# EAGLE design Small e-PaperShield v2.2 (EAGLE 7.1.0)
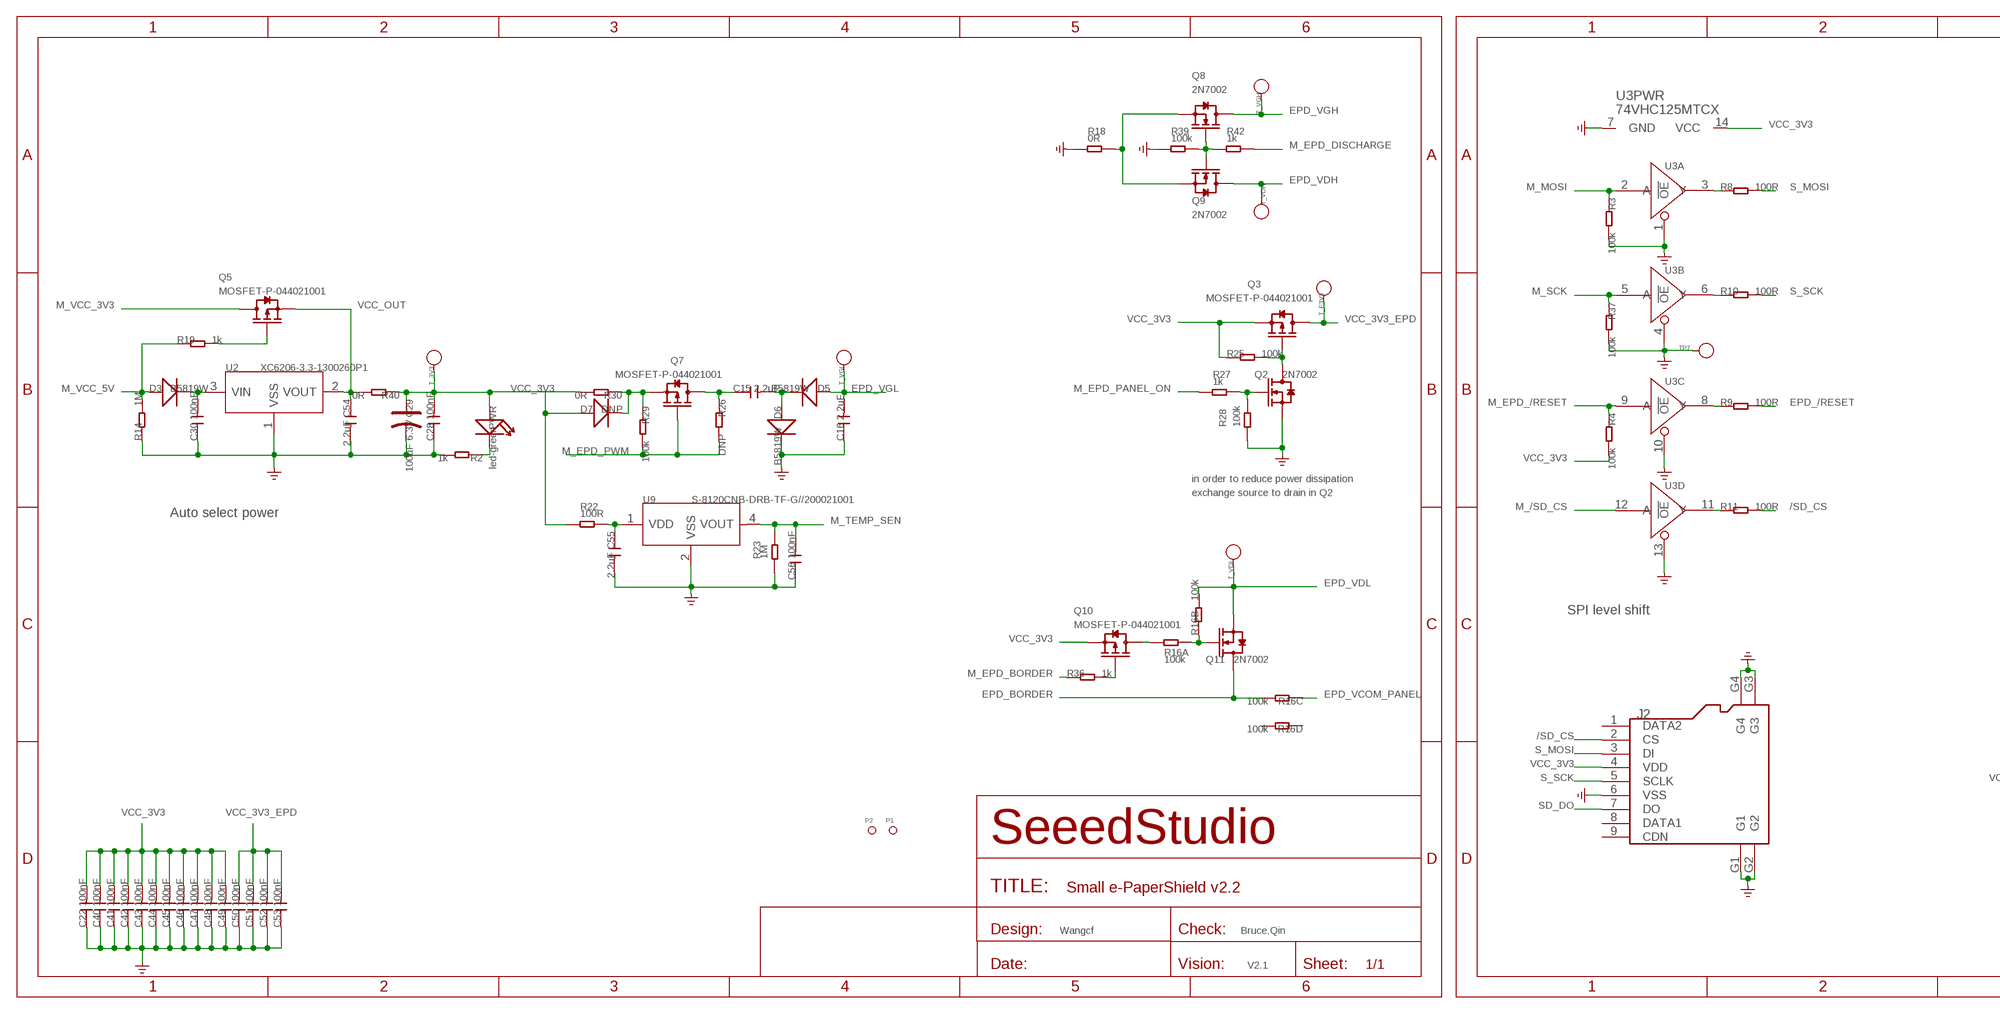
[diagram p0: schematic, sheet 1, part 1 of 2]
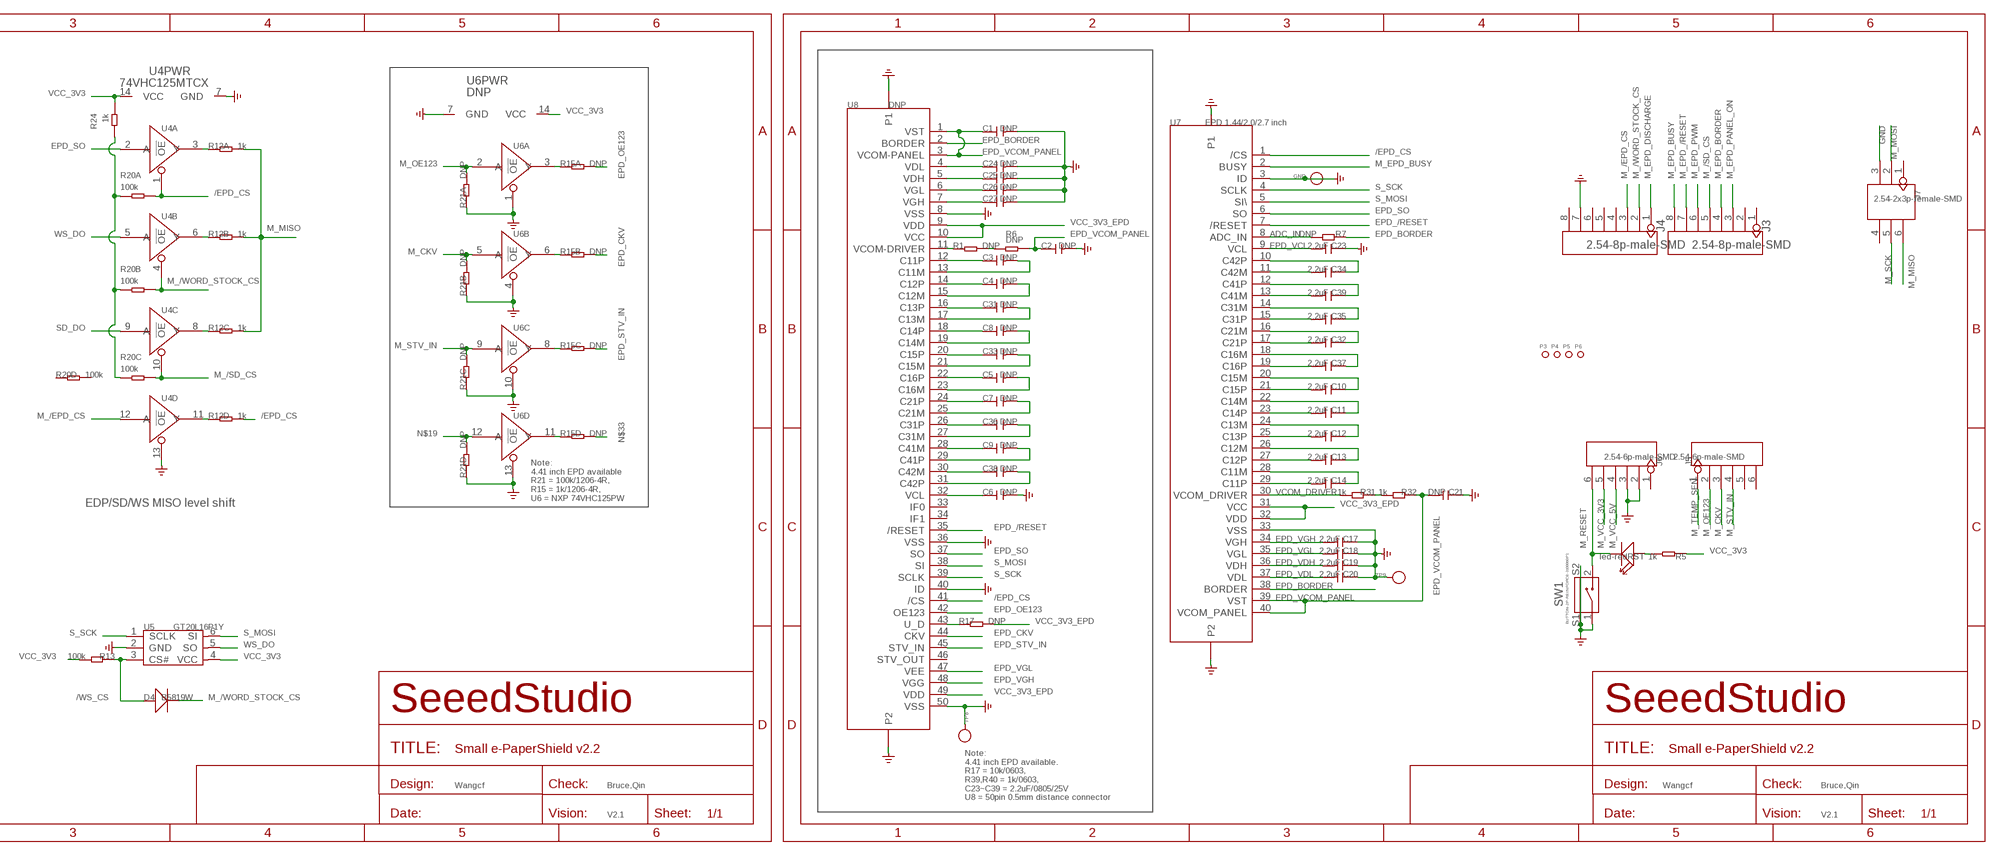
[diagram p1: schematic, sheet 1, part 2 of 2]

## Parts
C1  DNP  C-0805  [C0805]
C2  DNP  C-0805  [C0805]
C3  DNP  C-0805  [C0805]
C4  DNP  C-0805  [C0805]
C5  DNP  C-0805  [C0805]
C6  DNP  C-0805  [C0805]
C7  DNP  C-0805  [C0805]
C8  DNP  C-0805  [C0805]
C9  DNP  C-0805  [C0805]
C10  2.2uF  C-0805  [C0805]
C11  2.2uF  C-0805  [C0805]
C12  2.2uF  C-0805  [C0805]
C13  2.2uF  C-0805  [C0805]
C14  2.2uF  C-0805  [C0805]
C15  2.2uF  C-0805  [C0805]
C16  2.2uF  C-0805  [C0805]
C17  2.2uF  C-0805  [C0805]
C18  2.2uF  C-0805  [C0805]
C19  2.2uF  C-0805  [C0805]
C20  2.2uF  C-0805  [C0805]
C21  DNP  C-0805  [C0805]
C22  100nF  C-0603  [C0603]
C23  2.2uF  C-0805  [C0805]
C24  DNP  C-0805  [C0805]
C25  DNP  C-0805  [C0805]
C26  DNP  C-0805  [C0805]
C27  DNP  C-0805  [C0805]
C28  100nF  C-0603  [C0603]
C29  100uF 6.3V  CAP-AVX-B  [AVX-B]
C30  100nF  C-0603  [C0603]
C31  DNP  C-0805  [C0805]
C32  2.2uF  C-0805  [C0805]
C33  DNP  C-0805  [C0805]
C34  2.2uF  C-0805  [C0805]
C35  2.2uF  C-0805  [C0805]
C36  DNP  C-0805  [C0805]
C37  2.2uF  C-0805  [C0805]
C38  DNP  C-0805  [C0805]
C39  2.2uF  C-0805  [C0805]
C40  100nF  C-0603  [C0603]
C41  100nF  C-0603  [C0603]
C42  100nF  C-0603  [C0603]
C43  100nF  C-0603  [C0603]
C44  100nF  C-0603  [C0603]
C45  100nF  C-0603  [C0603]
C46  100nF  C-0603  [C0603]
C47  100nF  C-0603  [C0603]
C48  100nF  C-0603  [C0603]
C49  100nF  C-0603  [C0603]
C50  100nF  C-0603  [C0603]
C51  100nF  C-0603  [C0603]
C52  100nF  C-0603  [C0603]
C53  100nF  C-0603  [C0603]
C54  2.2uF  C-0805  [C0805]
C55  2.2uF  C-0805  [C0805]
C56  100nF  C-0603  [C0603]
D3  B5819W  D'1206'  [SOD123]
D4  B5819W  D'1206'  [SOD123]
D5  B5819W  D'1206'  [SOD123]
D6  B5819W  D'1206'  [SOD123]
D7  DNP  D'1206'  [SOD123]
GND  PAD-TEST-POINT'3535'  [TP_3535]
J2  HOLDER-MICROSD-9P  [9P-SMD-W/-RING]
J3  2.54-8p-male-SMD  HEADER-8P-2.54-SMD  [8P-2.54-SMD]
J4  2.54-8p-male-SMD  HEADER-8P-2.54-SMD  [8P-2.54-SMD]
J5  2.54-6p-male-SMD  HEADER-6P-SMD  [6P-2.54-SMD]
J6  2.54-6p-male-SMD  HEADER-6P-SMD  [6P-2.54-SMD]
J7  2.54-2x3p-female-SMD  HEADER-2X3P-SMD  [2X3P-2.54-SMD]
P1  PAD-MARK'ANNULAR'  [ROUND-MARK-1.0]
P2  PAD-MARK'ANNULAR'  [ROUND-MARK-1.0]
P3  PAD-MARK'ANNULAR'  [ROUND-MARK-1.0]
P4  PAD-MARK'ANNULAR'  [ROUND-MARK-1.0]
P5  PAD-MARK'ANNULAR'  [ROUND-MARK-1.0]
P6  PAD-MARK'ANNULAR'  [ROUND-MARK-1.0]
PWR  led-green  LED'RIGHT'  [LED-SIDE-VIEW-0603-RIGHT]
Q2  2N7002  MOSFET-N'SOT23'  [SOT23]
Q3  MOSFET-P-044021001  [SOT23]
Q5  MOSFET-P-044021001  [SOT23]
Q7  MOSFET-P-044021001  [SOT23]
Q8  2N7002  MOSFET-N'SOT23'  [SOT23]
Q9  2N7002  MOSFET-N'SOT23'  [SOT23]
Q10  MOSFET-P-044021001  [SOT23]
Q11  2N7002  MOSFET-N'SOT23'  [SOT23]
R1  DNP  R-0603  [R0603]
R2  1k  R-0603  [R0603]
R3  100k  R-0603  [R0603]
R4  100k  R-0603  [R0603]
R5  1k  R-0603  [R0603]
R6  DNP  R-0603  [R0603]
R7  DNP  R-0603  [R0603]
R8  100R  R-0603  [R0603]
R9  100R  R-0603  [R0603]
R10  100R  R-0603  [R0603]
R11  100R  R-0603  [R0603]
R12  1k  R-4R-1206  [1206-8-3.3X2.4]
R13  100k  R-0603  [R0603]
R14  1M  R-0603  [R0603]
R15  DNP  R-4R-1206  [1206-8-3.3X2.4]
R16  100k  R-4R-1206  [1206-8-3.3X2.4]
R17  DNP  R-0603  [R0603]
R18  0R  R-0603  [R0603]
R19  1k  R-0603  [R0603]
R20  100k  R-4R-1206  [1206-8-3.3X2.4]
R21  DNP  R-4R-1206  [1206-8-3.3X2.4]
R22  100R  R-0603  [R0603]
R23  1M  R-0603  [R0603]
R24  1k  R-0603  [R0603]
R25  100k  R-0603  [R0603]
R26  DNP  R-0603  [R0603]
R27  1k  R-0603  [R0603]
R28  100k  R-0603  [R0603]
R29  100k  R-0603  [R0603]
R30  0R  R-0603  [R0603]
R31  1k  R-0603  [R0603]
R32  1k  R-0603  [R0603]
R36  1k  R-0603  [R0603]
R37  100k  R-0603  [R0603]
R39  100k  R-0603  [R0603]
R40  0R  R-0603  [R0603]
R42  1k  R-0603  [R0603]
RST  led-red  LED'RIGHT'  [LED-SIDE-VIEW-0603-RIGHT]
SW1  BUTTON-2P-REINFORCE-3100060P1  [4P-SMD-7.0X3.5X3.5H-90D]
T_3V3  PAD-TEST-POINT'3535'  [TP_3535]
T_E3V3  PAD-TEST-POINT'3535'  [TP_3535]
T_VDH  PAD-TEST-POINT'3535'  [TP_3535]
T_VDL  PAD-TEST-POINT'3535'  [TP_3535]
T_VGH  PAD-TEST-POINT'3535'  [TP_3535]
T_VGL  PAD-TEST-POINT'3535'  [TP_3535]
TP7  PAD-TEST-POINT'3535'  [TP_3535]
TP8  PAD-TEST-POINT'3535'  [TP_3535]
TP9  PAD-TEST-POINT'3535'  [TP_3535]
U2  XC6206-3.3-1300260P1  [SOT23]
U3  74VHC125MTCX  74VHC125PW  [TSSOP14]
U4  74VHC125MTCX  74VHC125PW  [TSSOP14]
U5  GT20L16P1Y  [SOT23-6]
U6  DNP  74VHC125PW  [TSSOP14]
U7  EPD 1.44/2.0/2.7 inch  TFT-EPD-PANEL  [40P-0.5]
U8  DNP  TFT-EPD-PANEL  [50P-0.5]
U9  S-8120CNB-DRB-TF-G//200021001  S-8110C/8120C  [SC-82AB]

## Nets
3V3_LOG: R20.1 R20.2 R20.3 R24.2
/EPD_CS: R12.5 R20.8 U4.1(A:!OE) U7.1(/CS) U8.41(/CS)
/SD_CS: J2.2(CS) R11.2
/WS_CS: D4.+ R13.1 U5.3(CS#)
ADC_IN: R7.2 U7.8(ADC_IN)
EPD_/RESET: R9.2 U7.7(/RESET) U8.35(/RESET)
EPD_BORDER: Q11.3(D) R7.1 R16.6 U7.38(BORDER) U8.2(BORDER)
EPD_CKV: R15.7 U8.44(CKV)
EPD_OE123: R15.8 U8.42(OE123)
EPD_SO: U4.2(A:A) U7.6(SO) U8.37(SO)
EPD_STV_IN: R15.6 U8.45(STV_IN)
EPD_VCL: C23.2 U7.9(VCL)
EPD_VCOM_PANEL: C1.1 C2.1 C21.2 R6.2 R16.3 R32.1 U7.39(VST) U7.40(VCOM_PANEL) U8.1(VST) U8.3(VCOM-PANEL)
EPD_VDH: C19.2 C25.1 Q9.3(D) T_VDH.T U7.36(VDH) U8.5(VDH)
EPD_VDL: C20.2 C24.1 Q11.2(S) R16.7 T_VDL.T U7.37(VDL) U8.4(VDL)
EPD_VGH: C17.2 C27.1 Q8.3(D) T_VGH.T U7.34(VGH) U8.7(VGH) U8.48(VGG)
EPD_VGL: C16.2 C18.2 C26.1 D5.+ T_VGL.T U7.35(VGL) U8.6(VGL) U8.47(VEE)
GND: C1.2 C2.2 C6.2 C16.1 C17.1 C18.1 C19.1 C20.1 C21.1 C22.1 C23.1 C24.2 C25.2 C26.2 C27.2 C28.1 C29.- C30.1 C40.1 C41.1 C42.1 C43.1 C44.1 C45.1 C46.1 C47.1 C48.1 C49.1 C50.1 C51.1 C52.1 C53.1 C54.2 C55.2 C56.1 D6.- GND.T J2.6(VSS) J2.G1 J2.G2 J2.G3 J2.G4 J4.7 J6.2 J6.3 J7.3 Q2.2(S) R2.2 R3.2 R14.1 R18.1 R21.1 R21.2 R21.3 R21.4 R23.1 R28.1 R37.2 R39.1 SW1.1 SW1.S1 SW1.S2 TP7.T TP8.T TP9.T U2.1(VSS) U3.1(A:!OE) U3.4(B:!OE) U3.7(PWR:GND) U3.10(C:!OE) U3.13(D:!OE) U4.7(PWR:GND) U4.13(D:!OE) U5.2(GND) U6.1(A:!OE) U6.4(B:!OE) U6.7(PWR:GND) U6.10(C:!OE) U6.13(D:!OE) U7.3(ID) U7.33(VSS) U7.P1 U7.P2 U8.8(VSS) U8.36(VSS) U8.40(ID) U8.50(VSS) U8.P1 U8.P2 U9.2(VSS)
M_/EPD_CS: J4.3 U4.12(D:A)
M_/SD_CS: J3.5 R20.6 U3.12(D:A) U4.10(C:!OE)
M_/WORD_STOCK_CS: D4.- J4.2 R20.7 U4.4(B:!OE)
M_CKV: J5.3 R21.7 U6.5(B:A)
M_EPD_/RESET: J3.7 R4.1 U3.9(C:A)
M_EPD_BORDER: J3.4 R36.1
M_EPD_BUSY: J3.8 U7.2(BUSY)
M_EPD_DISCHARGE: J4.1 R42.2
M_EPD_PANEL_ON: J3.3 R27.1
M_EPD_PWM: J3.6 Q7.1(G) R26.2 R29.2
M_MISO: J7.6 R12.6 R12.7 R12.8
M_MOSI: J7.2 R3.1 U3.2(A:A)
M_OE123: J5.2 R21.8 U6.2(A:A)
M_RESET: J6.6 RST.2(-) SW1.2
M_SCK: J7.5 R37.1 U3.5(B:A)
M_STV_IN: J5.4 R21.6 U6.9(C:A)
M_TEMP_SEN: C56.2 J5.1 R23.2 U9.4(VOUT)
M_VCC_3V3: J6.5 Q5.3(D)
M_VCC_5V: D3.+ J6.4 R14.2 R19.1
N$1: PWR.2(-) R2.1
N$2: Q5.1(G) R19.2
N$3: C15.2 D5.- D6.+
N$4: D7.- Q7.2(S) R29.1 R30.1
N$6: Q2.1(G) R27.2 R28.2
N$7: R11.1 U3.11(D:Y)
N$8: C30.2 D3.- U2.3(VIN)
N$9: C15.1 Q7.3(D) R26.1
N$10: Q8.1(G) Q9.1(G) R39.2 R42.1
N$11: Q2.3(D) Q3.1(G) R25.2
N$12: R31.1 R32.2
N$13: Q10.3(D) R16.1
N$14: Q10.1(G) R36.2
N$15: C4.1 U8.14(C12P)
N$16: Q8.2(S) Q9.2(S) R18.2
N$19: R21.5 U6.12(D:A)
N$20: R12.1 U4.3(A:Y)
N$21: R12.2 U4.6(B:Y)
N$22: R12.3 U4.8(C:Y)
N$23: R15.1 U6.3(A:Y)
N$24: R15.3 U6.8(C:Y)
N$25: R15.4 U6.11(D:Y)
N$26: R15.2 U6.6(B:Y)
N$27: R12.4 U4.11(D:Y)
N$28: Q11.1(G) R16.2 R16.8
N$30: R1.2 R6.1
N$33: R15.5
N$34: C34.1 U7.10(C42P)
N$35: C34.2 U7.11(C42M)
N$36: C39.1 U7.12(C41P)
N$37: C39.2 U7.13(C41M)
N$39: C4.2 U8.15(C12M)
N$40: C3.1 U8.12(C11P)
N$41: C31.2 U8.17(C13M)
N$42: C31.1 U8.16(C13P)
N$43: C8.1 U8.18(C14P)
N$44: C8.2 U8.19(C14M)
N$45: C33.2 U8.21(C15M)
N$46: C33.1 U8.20(C15P)
N$47: C5.1 U8.22(C16P)
N$48: C5.2 U8.23(C16M)
N$49: C7.1 U8.24(C21P)
N$50: C7.2 U8.25(C21M)
N$51: C36.1 U8.26(C31P)
N$52: C36.2 U8.27(C31M)
N$53: C9.1 U8.28(C41M)
N$54: C9.2 U8.29(C41P)
N$55: C38.1 U8.30(C42M)
N$56: C38.2 U8.31(C42P)
N$57: C6.1 U8.32(VCL)
N$58: R1.1 U8.11(VCOM-DRIVER)
N$67: R17.1 U8.43(U_D)
N$74: R8.1 U3.3(A:Y)
N$76: R10.1 U3.6(B:Y)
N$80: R9.1 U3.8(C:Y)
N$81: C35.1 U7.14(C31M)
N$82: C3.2 U8.13(C11M)
N$85: C35.2 U7.15(C31P)
N$87: R5.2 RST.1(+)
N$88: C32.1 U7.16(C21M)
N$89: C32.2 U7.17(C21P)
N$90: C37.1 U7.18(C16M)
N$91: C37.2 U7.19(C16P)
N$92: C10.1 U7.20(C15M)
N$93: C10.2 U7.21(C15P)
N$94: C11.1 U7.22(C14M)
N$95: C11.2 U7.23(C14P)
N$96: C12.1 U7.24(C13M)
N$97: C12.2 U7.25(C13P)
N$98: C13.1 U7.26(C12M)
N$99: C13.2 U7.27(C12P)
N$100: C14.1 U7.28(C11M)
N$101: C14.2 U7.29(C11P)
S_MOSI: J2.3(DI) R8.2 U5.6(SI) U7.5(SI\) U8.38(SI)
S_SCK: J2.5(SCLK) R10.2 U5.1(SCLK) U7.4(SCLK) U8.39(SCLK)
SD_DO: J2.7(DO) U4.9(C:A)
VCC_3V3: C22.2 C28.2 C29.+ C40.2 C41.2 C42.2 C43.2 C44.2 C45.2 C46.2 C47.2 C48.2 C49.2 D7.+ J2.4(VDD) PWR.1(+) Q3.2(S) Q10.2(S) R4.2 R5.1 R13.2 R22.1 R24.1 R25.1 R30.2 R40.1 T_3V3.T U3.14(PWR:VCC) U4.14(PWR:VCC) U5.4(VCC) U6.14(PWR:VCC)
VCC_3V3_EPD: C50.2 C51.2 C52.2 C53.2 Q3.3(D) R17.2 T_E3V3.T U7.31(VCC) U7.32(VDD) U8.9(VDD) U8.10(VCC) U8.49(VDD)
VCC_OUT: C54.1 Q5.2(S) R40.2 U2.2(VOUT)
VCOM_DRIVER: R31.2 U7.30(VCOM_DRIVER)
VDD: C55.1 R22.2 U9.1(VDD)
WS_DO: U4.5(B:A) U5.5(SO)
Unconnected: J2.1(DATA2) J2.8(DATA1) J2.9(CDN) J3.1 J3.2 J4.4 J4.5 J4.6 J4.8 J5.5 J5.6 J6.1 J7.1 J7.4 R16.4 R16.5 R20.4 R20.5 U8.33(IF0) U8.34(IF1) U8.46(STV_OUT)

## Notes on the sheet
- in order to reduce power dissipation
- exchange source to drain in Q2
- Auto select power
- Note:
  4.41 inch EPD available
  R21 = 100k/1206-4R,
  R15 = 1k/1206-4R,
  U6 = NXP 74VHC125PW
- EDP/SD/WS MISO level shift
- SPI level shift
- Wangcf | Bruce,Qin | Wangcf | Bruce,Qin | Wangcf | Bruce,Qin
- Note:
  4.41 inch EPD available.
  R17 = 10k/0603, 
  R39,R40 = 1k/0603, 
  C23~C39 = 2.2uF/0805/25V
  U8 = 50pin 0.5mm distance connector
- V2.1 | V2.1 | V2.1

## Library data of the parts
C1-C28 C30-C56 = Discrete:C*: Ceramic Capacitors
C29 = Discrete:CAP*: Electrolytic Capacitors,Tantalum Capacitors and Super Capacitors
D3-D7 = Discrete:D*
GND T_3V3 T_E3V3 T_VDH T_VDL T_VGH T_VGL TP7-TP9 = Discrete:PAD-TEST-POINT; PARTNO: DNP
J2 = Connector :HOLDER-MICROSD-9P
J3 J4 = Connector:HEADER-8P
J5 J6 = Connector:HEADER-6P
J7 = Connector:HEADER-2X3P
P1-P6 = Discrete:PAD-MARK; PARTNO: DNP
PWR RST = Discrete:LED*
Q2 Q8 Q9 Q11 = Discrete:MOSFET-N: IRLL014: http://www.vishay.com/docs/91319/sihll014.pdf
Q3 Q5 Q7 Q10 = OPL:MOSFET-P: CJ2305：SMD MOSFET P-CH 8V-4.1A
R1-R11 R13 R14 R17-R19 R22-R32 R36 R37 R39 R40 R42 = Discrete:R*
R12 R15 R16 R20 R21 = Discrete:R-4R*: Resistor Array
SW1 = Discrete:BUTTON-2P-REINFORCE: TS-1188E http://www.best-dz.com/?thread-374-2.html SMD Button
U2 = OPL:XC6206-3.3: LOW ESR Cap.Compatible Positive Voltage Regulators
U3 U4 U6 = IC:74V*125: Quad Buffer/Line Driver;3-state
U5 = template:GT20L16P1Y
U7 = moudle:TFT-EPD-PANEL: 1.44inch/2.0inch/2.7inch TFT EPD Panel
U8 = template:TFT-EPD-PANEL: 4.4inch TFT EPD PANEL
U9 = template:S-8110C/8120C: COMS Temperature Sensor IC

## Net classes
0 default: width 0.152 mm, drill 0.305 mm, clearance 0.152 mm

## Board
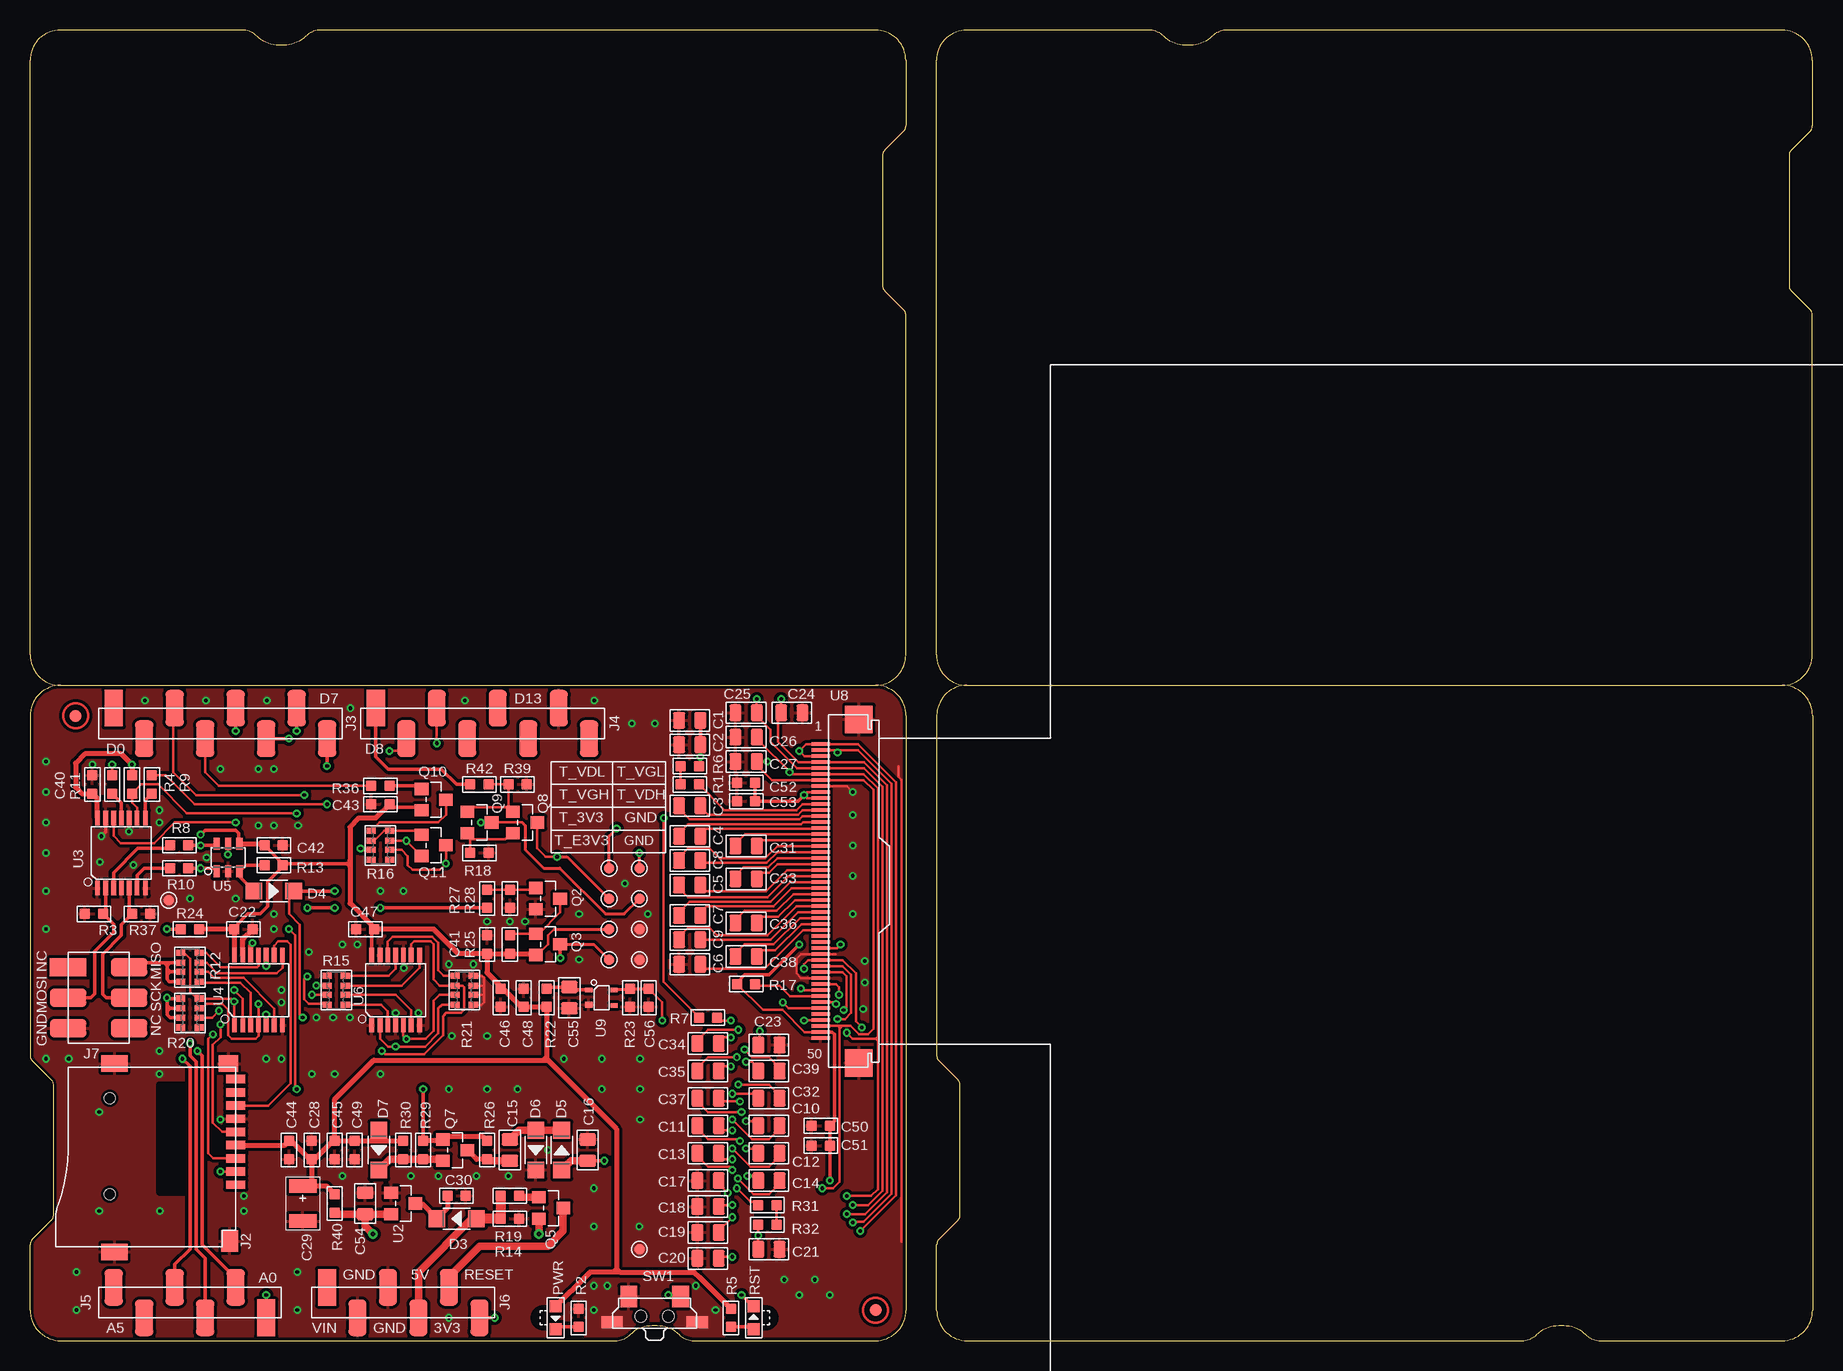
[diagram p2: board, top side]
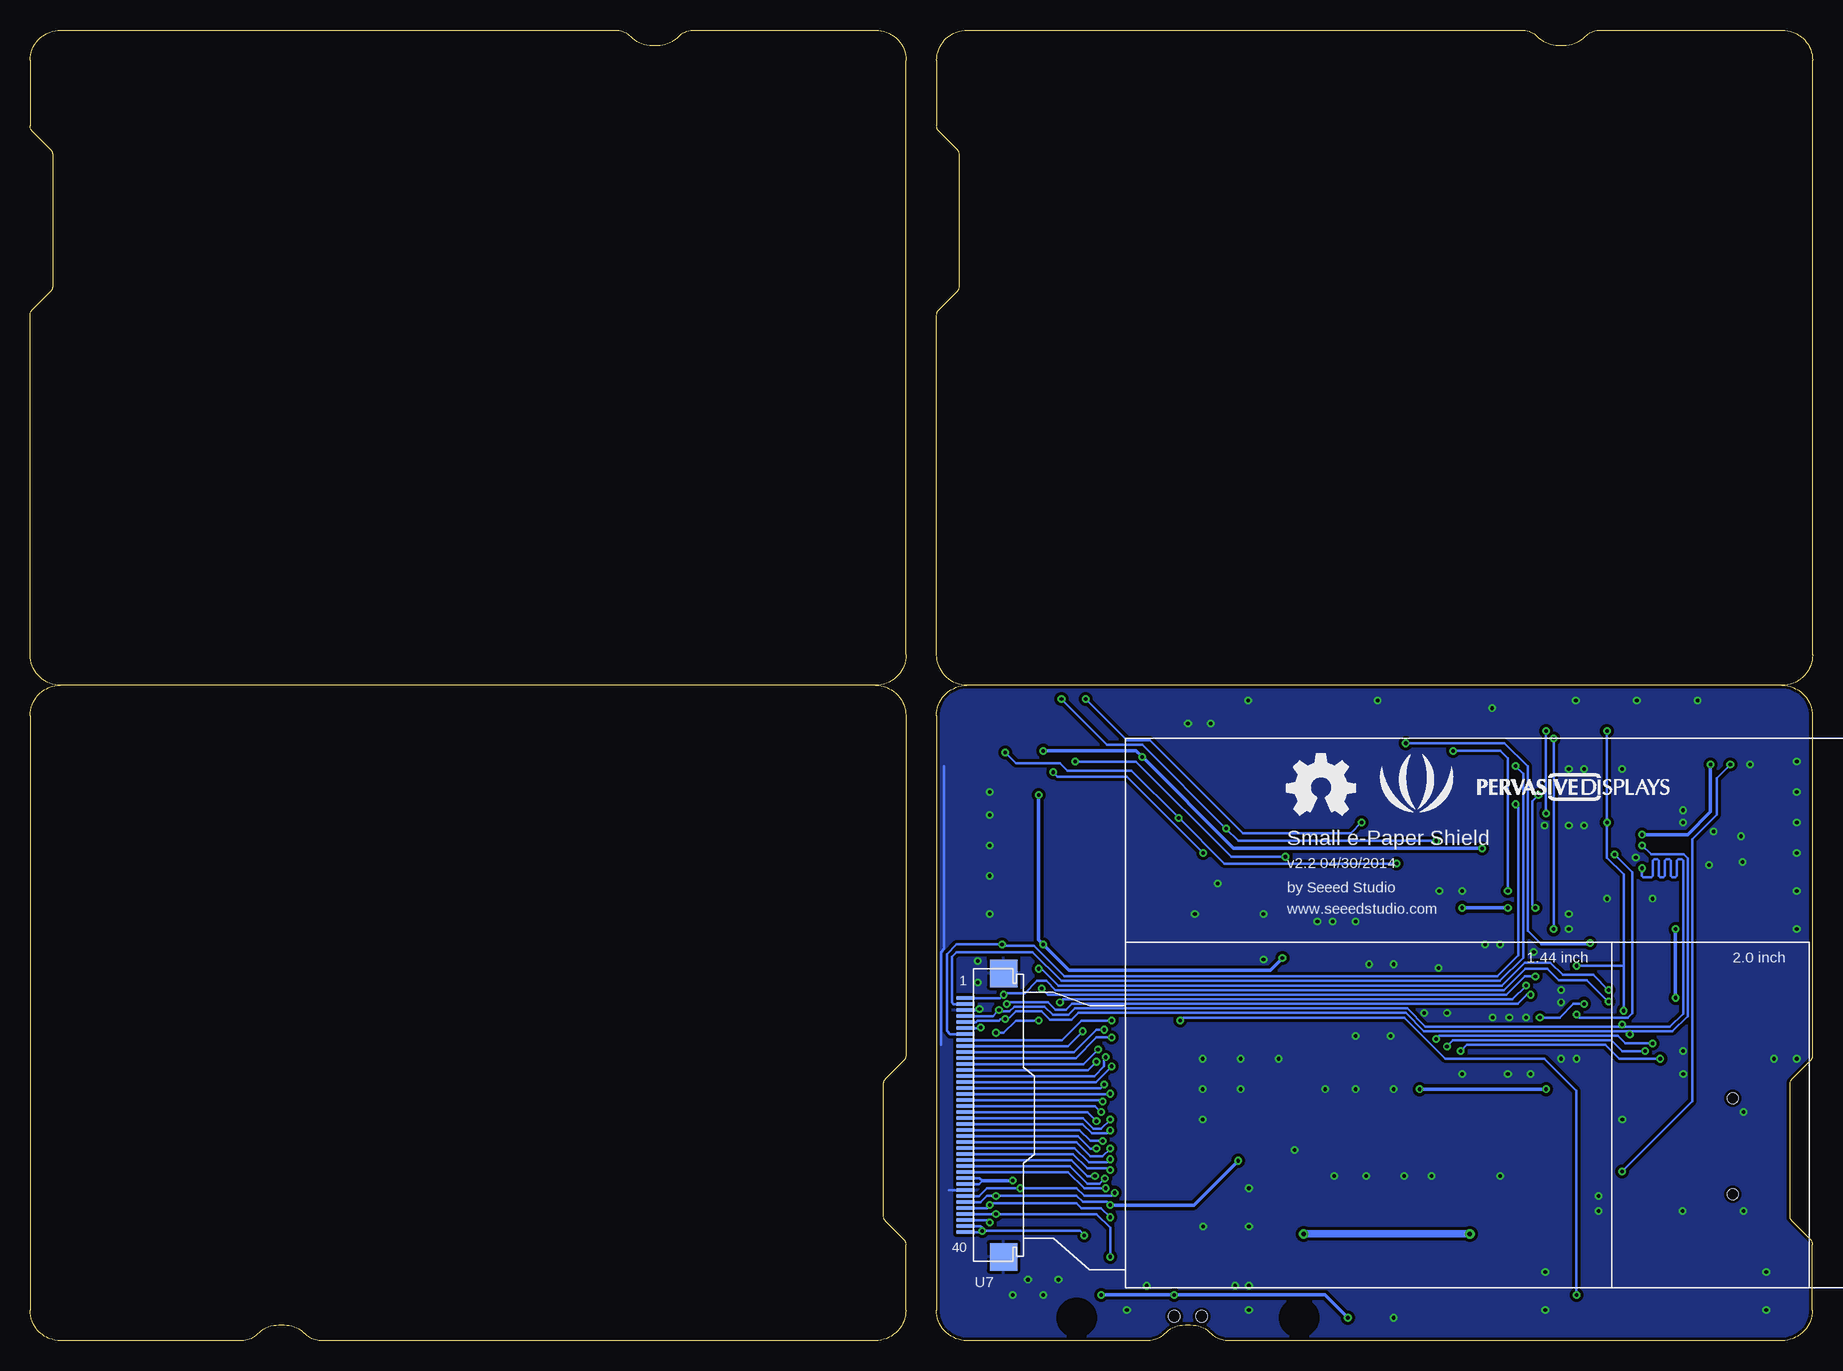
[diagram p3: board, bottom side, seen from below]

Size 148.59 x 109.22 mm. Coordinates in mm from the lower left corner, seen from the top.
Outline: 86 segments
Copper layers (1*16): Top 0.035mm / dielectric 1.5mm / Bottom 0.035mm
Design rules "SeeedStudio_2layer_DRU_no_angle_20140221 *": minimum track width 6mil, minimum drill 12mil, track to track 6mil, track to pad 6mil, pad to pad 6mil, via to via 6mil, smd to smd 0mil, copper to edge 10mil, drill to drill 10mil, minimum pad ring 10mil, minimum via ring 6mil, stop-mask expansion 2mil, vias tented up to drill 100mil, thermal gap 10mil
Holes 2.03 mm at 7.62,113.66 140.97,113.66 140.97,-4.45 7.62,-4.45
tRestrict: area 36.7,29.9 to 37.2,30.1; area 36.7,29.9 to 37.2,30.1; area 36.7,29.1 to 37.2,29.3; area 36.6,28.3 to 37.3,28.5; area 42,1.1 to 43.6,2.7; area 60.5,1.1 to 62.1,2.7
bRestrict: area 41.4,0.5 to 44.2,3.3; area 59.9,0.5 to 62.8,3.3

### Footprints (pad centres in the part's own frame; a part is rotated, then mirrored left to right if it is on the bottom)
C0805 = smd 1.016 x 1.397: 1 -0.889,0; 2 0.889,0
C0603 = smd 0.889 x 0.889: 1 -0.762,0; 2 0.762,0
AVX-B = smd 1.143 x 2.286: + -1.46,0; - 1.46,0
SOD123 = smd 1.397 x 1.397: + -1.651,0; - 1.651,0
TP_3535 = smd 0.889 x 0.889: T 0,0
9P-SMD-W/-RING = smd 1.6 x 0.7: 1 0,2.25; 2 0,1.15; 3 0,0.05; 4 0,-1.05; 5 0,-2.15; 6 0,-3.25; 7 0,-4.35; 8 0,-5.45; 9 0,-6.55 | smd 1.6 x 1.4: G1 0.6,-7.85 | smd 2.2 x 1.4: G2 10.1,-7.85; G3 10.1,7.85 | smd 1.4 x 1.8: G4 0.5,6.95 | hole 0.9: 10.5,-4.95; 10.5,3.05
8P-2.54-SMD = smd 3.048 x 1.524: 1 1.27,8.89; 2 -1.27,6.35; 3 1.27,3.81; 4 -1.27,1.27; 5 1.27,-1.27; 6 -1.27,-3.81; 7 1.27,-6.35; 8 -1.27,-8.89
6P-2.54-SMD = smd 3.048 x 1.524: 1 1.27,6.35; 2 -1.27,3.81; 3 1.27,1.27; 4 -1.27,-1.27; 5 1.27,-3.81; 6 -1.27,-6.35
2X3P-2.54-SMD = smd 3.048 x 1.524: 1 -2.54,2.54; 2 -2.54,0; 3 -2.54,-2.54; 4 2.54,-2.54; 5 2.54,0; 6 2.54,2.54
ROUND-MARK-1.0 = smd 1.016 x 1.016: P$1 0,0
LED-SIDE-VIEW-0603-RIGHT = smd 1 x 1: 1 0,-0.95; 2 0,0.95
SOT23 = smd 1.016 x 1.143: 1 -0.889,-1.016; 2 0.889,-1.016; 3 0,1.016
R0603 = smd 0.889 x 0.889: 1 -0.762,0; 2 0.762,0
1206-8-3.3X2.4 = smd 0.508 x 0.762: 1 -1.206,-0.762; 2 -0.381,-0.762; 3 0.381,-0.762; 4 1.206,-0.762; 5 1.206,0.762; 6 0.381,0.762; 7 -0.381,0.762; 8 -1.206,0.762
4P-SMD-7.0X3.5X3.5H-90D = smd 1.397 x 1.778: 1 -2.159,1.651; 2 2.159,1.651 | smd 1.778 x 1.016: S1 -3.556,-0.508; S2 3.556,-0.508 | hole 0.95: -1.15,0; 1.15,0
TSSOP14 = smd 0.4 x 1.2: 1 -2,-2.925; 2 -1.3,-2.925; 3 -0.65,-2.925; 4 0,-2.925; 5 0.65,-2.925; 6 1.3,-2.925; 7 2,-2.925; 8 2,2.925; 9 1.3,2.925; 10 0.65,2.925; 11 0,2.925; 12 -0.65,2.925; 13 -1.3,2.925; 14 -2,2.925
SOT23-6 = smd 0.508 x 1.016: 1 -0.95,-1.143; 2 0,-1.143; 3 0.95,-1.143; 4 0.95,1.143; 5 0,1.143; 6 -0.95,1.143
40P-0.5 = smd 1.524 x 0.305: 1 -0.762,9.75; 2 -0.762,9.25; 3 -0.762,8.75; 4 -0.762,8.25; 5 -0.762,7.75; 6 -0.762,7.25; 7 -0.762,6.75; 8 -0.762,6.25; 9 -0.762,5.75; 10 -0.762,5.25; 11 -0.762,4.75; 12 -0.762,4.25; 13 -0.762,3.75; 14 -0.762,3.25; 15 -0.762,2.75; 16 -0.762,2.25; 17 -0.762,1.75; 18 -0.762,1.25; 19 -0.762,0.75; 20 -0.762,0.25; 21 -0.762,-0.25; 22 -0.762,-0.75; 23 -0.762,-1.25; 24 -0.762,-1.75; 25 -0.762,-2.25; 26 -0.762,-2.75; 27 -0.762,-3.25; 28 -0.762,-3.75; 29 -0.762,-4.25; 30 -0.762,-4.75; 31 -0.762,-5.25; 32 -0.762,-5.75; 33 -0.762,-6.25; 34 -0.762,-6.75; 35 -0.762,-7.25; 36 -0.762,-7.75; 37 -0.762,-8.25; 38 -0.762,-8.75; 39 -0.762,-9.25; 40 -0.762,-9.75 | smd 2.286 x 2.286: P1 2.413,11.811; P2 2.413,-11.811
50P-0.5 = smd 1.524 x 0.305: 1 -0.762,12.25; 2 -0.762,11.75; 3 -0.762,11.25; 4 -0.762,10.75; 5 -0.762,10.25; 6 -0.762,9.75; 7 -0.762,9.25; 8 -0.762,8.75; 9 -0.762,8.25; 10 -0.762,7.75; 11 -0.762,7.25; 12 -0.762,6.75; 13 -0.762,6.25; 14 -0.762,5.75; 15 -0.762,5.25; 16 -0.762,4.75; 17 -0.762,4.25; 18 -0.762,3.75; 19 -0.762,3.25; 20 -0.762,2.75; 21 -0.762,2.25; 22 -0.762,1.75; 23 -0.762,1.25; 24 -0.762,0.75; 25 -0.762,0.25; 26 -0.762,-0.25; 27 -0.762,-0.75; 28 -0.762,-1.25; 29 -0.762,-1.75; 30 -0.762,-2.25; 31 -0.762,-2.75; 32 -0.762,-3.25; 33 -0.762,-3.75; 34 -0.762,-4.25; 35 -0.762,-4.75; 36 -0.762,-5.25; 37 -0.762,-5.75; 38 -0.762,-6.25; 39 -0.762,-6.75; 40 -0.762,-7.25; 41 -0.762,-7.75; 42 -0.762,-8.25; 43 -0.762,-8.75; 44 -0.762,-9.25; 45 -0.762,-9.75; 46 -0.762,-10.25; 47 -0.762,-10.75; 48 -0.762,-11.25; 49 -0.762,-11.75; 50 -0.762,-12.25 | smd 2.286 x 2.286: P1 2.413,14.311; P2 2.413,-14.311
SC-82AB = smd 0.4 x 0.6: 1 -0.65,-1.05; 3 0.65,1.05; 4 -0.65,1.05 | smd 0.5 x 0.6: 2 0.6,-1.05

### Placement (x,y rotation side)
C1  54.99,51.69 180 top
C2  54.99,49.66 180 top
C3  54.99,44.58 180 top
C4  54.99,42.04 0 top
C5  54.99,37.97 180 top
C6  54.99,31.37 180 top
C7  54.99,35.43 0 top
C8  54.99,40 0 top
C9  54.99,33.4 0 top
C10  61.59,17.91 0 top
C11  56.52,17.91 180 top
C12  61.59,15.62 0 top
C13  56.52,15.62 180 top
C14  61.59,13.33 0 top
C15  40,15.88 90 top
C16  46.48,15.88 270 top
C17  56.52,13.33 0 top
C18  56.52,11.18 0 top
C19  56.52,9.02 0 top
C20  56.52,6.86 0 top
C21  61.59,7.62 180 top
C22  17.78,34.29 180 top
C23  61.59,24.64 180 top
C24  63.5,52.32 0 top
C25  59.69,52.32 180 top
C26  59.69,50.29 180 top
C27  59.69,48.26 180 top
C28  23.49,15.88 270 top
C29  22.73,11.43 270 top
C30  35.56,12.06 180 top
C31  59.69,41.21 0 top
C32  61.59,20.19 180 top
C33  59.69,38.48 0 top
C34  56.52,24.77 0 top
C35  56.52,22.48 0 top
C36  59.69,34.8 0 top
C37  56.52,20.19 180 top
C38  59.69,32 0 top
C39  61.59,22.48 180 top
C40  5.21,46.36 270 top
C41  38.1,33.02 270 top
C42  20.32,41.27 180 top
C43  29.21,44.7 0 top
C44  21.59,15.88 90 top
C45  25.4,15.88 90 top
C46  39.24,28.57 90 top
C47  27.94,34.29 0 top
C48  41.15,28.57 270 top
C49  27.05,15.88 90 top
C50  65.91,17.91 0 top
C51  65.91,16.26 0 top
C52  59.69,46.48 0 top
C53  59.69,44.96 0 top
C54  27.94,11.43 90 top
C55  44.96,28.57 270 top
C56  51.56,28.57 90 top
D3  35.56,10.16 180 top
D4  20.32,37.47 0 top
D5  44.32,15.88 90 top
D6  42.16,15.88 270 top
D7  29.08,15.88 270 top
GND  50.8,31.75 0 top
J2  17.14,15.24 180 top
J3  15.88,51.44 90 top
J4  37.72,51.44 90 top
J5  13.34,3.18 270 top
J6  31.11,3.18 90 top
J7  5.71,28.57 0 top
P1  3.81,52.07 0 top
P2  70.48,2.54 0 top
P3  not placed on the board
P4  not placed on the board
P5  not placed on the board
P6  not placed on the board
PWR  43.81,1.91 180 top
Q2  43.18,36.83 270 top
Q3  43.18,33.02 270 top
Q5  43.43,11.05 270 top
Q7  35.43,15.88 270 top
Q8  41.27,43.18 270 top
Q9  37.46,43.18 270 top
Q10  33.66,45.09 270 top
Q11  33.66,41.27 270 top
R1  54.99,46.36 180 top
R2  45.72,1.91 90 top
R3  5.33,35.56 180 top
R4  8.51,46.36 90 top
R5  58.42,1.91 270 top
R6  54.99,47.88 0 top
R7  56.52,26.92 0 top
R8  12.45,41.27 0 top
R9  10.16,46.36 90 top
R10  12.45,39.37 0 top
R11  6.86,46.36 90 top
R12  13.34,31.11 90 top
R13  20.32,39.62 0 top
R14  40,10.16 180 top
R15  25.53,29.21 90 top
R16  29.21,41.27 270 top
R17  59.69,29.72 180 top
R18  37.46,40.64 180 top
R19  40,12.06 0 top
R20  13.34,27.3 270 top
R21  36.2,29.21 90 top
R22  43.05,28.57 90 top
R23  50.04,28.57 90 top
R24  13.34,34.29 180 top
R25  40,33.02 90 top
R26  38.1,15.88 90 top
R27  38.1,36.83 90 top
R28  40,36.83 90 top
R29  32.77,15.88 90 top
R30  31.11,15.88 90 top
R31  61.47,11.3 180 top
R32  61.47,9.65 0 top
R36  29.21,46.23 0 top
R37  9.27,35.56 0 top
R39  40.64,46.36 180 top
R40  25.4,11.43 270 top
R42  37.46,46.36 180 top
RST  60.32,1.91 0 top
SW1  52.07,2.03 0 top
T_3V3  48.26,34.29 90 top
T_E3V3  48.26,31.75 270 top
T_VDH  50.8,36.83 270 top
T_VDL  48.26,39.37 180 top
T_VGH  48.26,36.83 270 top
T_VGL  50.8,39.37 90 top
TP7  11.56,36.7 0 top
TP8  50.8,7.62 0 top
TP9  50.8,34.29 0 top
U2  31.11,11.43 270 top
U3  7.62,40.64 0 top
U4  19.05,29.21 0 top
U5  16.51,40.26 0 top
U6  30.48,29.21 0 top
U7  69.85,18.8 0 bottom
U8  66.67,37.47 0 top
U9  47.62,28.57 270 top
U$20  [LOGO_SILK]  33.02,45.72 0 bottom
U$47  [OSHW_FILLX200_NOTEXT]  43.81,43.81 0 bottom

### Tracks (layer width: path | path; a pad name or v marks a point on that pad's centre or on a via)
3V3_LOG  (via drill 0.3 pad 0.64)
  Top 0.305: R24.2 v11.43,34.29 | R20.1 11.49,28.51 v11.43,28.57 11.43,28.32 | R20.3 11.68,26.92 11.43,27.18 11.43,27.43 | 11.43,27.43 11.43,27.69 | 11.43,27.69 11.43,27.94 | 11.43,27.94 11.43,28.32 | R20.2 11.68,27.69 | 11.68,27.69 11.43,27.69 | 11.43,27.43 11.68,27.69 | 11.68,27.69 11.43,27.94 | 11.43,28.32 11.56,28.45
  Bottom 0.305: v11.43,34.29 v11.43,28.57
/EPD_CS  (via drill 0.3 pad 0.64)
  Top 0.203: R12.5 12.84,32.32 13.34,31.83 13.34,29.08 13.97,28.45 14.03,28.45 R20.8 16.76,28.51 v17.02,28.26 17.02,26.32 U4.1 | U8.41 67.19,29.71 67.44,29.46 v67.44,28.83
  Bottom 0.203: U7.1 67.72,28.55 v67.44,28.83 67.31,28.96 65.66,28.96 64.64,29.97 63.88,29.97 63.12,29.21 25.72,29.21 23.94,30.99 22.1,30.99 21.16,30.05 18.81,30.05 v17.02,28.26
/SD_CS  (via drill 0.3 pad 0.64)
  Top 0.203: R11.2 v6.86,48.01 | J2.2 v15.88,14.09 v15.88,14.1
  Bottom 0.203: v6.86,48.01 8,46.86 8,43.81 10.03,41.78 10.03,19.94 v15.88,14.1
/WS_CS
  Top 0.305: R13.1 17.97,39.62 U5.3 17.46,38.67 D4.+
ADC_IN  (via drill 0.3 pad 0.64)
  Top 0.203: v58.42,26.67 57.4,26.67 57.4,26.8 R7.2
  Bottom 0.203: U7.8 62.58,25.05 60.96,26.67 v58.42,26.67
EPD_/RESET  (via drill 0.3 pad 0.64)
  Top 0.203: U8.35 67.26,32.72 v67.56,33.02 | R9.2 11.3,47.12 13.72,44.7 v24.76,44.7
  Bottom 0.203: U7.7 71.88,25.55 72.16,25.83 72.16,32.2 71.34,33.02 v67.56,33.02 67.44,32.89 64.9,32.89 62.36,30.35 26.27,30.35 24.51,32.12 24.51,44.45 v24.76,44.7
EPD_BORDER  (via drill 0.3 pad 0.64)
  Top 0.203: U8.2 67.31,49.22 | 67.31,49.22 69.02,49.22 71.82,46.42 71.82,12.25 69.47,9.91 68.64,9.91 v68.58,9.84 | v67.31,49.02 67.31,49.22 | Q11.3 v34.67,39.75 34.16,39.24 31.88,39.24 31.5,39.62 31.5,40.39 30.99,40.89 R16.6 | R7.1 55.63,26.92 55.63,26.99 55.56,27.05 55.56,27.18 52.83,29.91 v52.83,43.56
  Bottom 0.203: U7.38 68.78,10.05 v68.58,9.84 | v34.67,39.75 49.02,39.75 v52.83,43.56 56.77,47.5 62.1,47.5 62.74,48.13 66.42,48.13 v67.31,49.02
EPD_CKV  (via drill 0.3 pad 0.64)
  Top 0.203: U8.44 67.03,28.21 v67.18,28.07 | R15.7 v23.49,28.83
  Bottom 0.203: v67.18,28.07 67.06,28.19 63.75,28.19 63.12,27.56 62.23,27.56 61.72,28.07 24.59,28.07 23.83,28.83 v23.49,28.83
EPD_OE123  (via drill 0.3 pad 0.64)
  Top 0.203: R15.8 24.7,28.07 23.24,28.07 22.86,28.45 22.86,30.1 v23.11,30.35 | U8.42 64.38,29.21 v64.26,29.34
  Bottom 0.203: v23.11,30.35 24,30.35 25.53,28.83 63.75,28.83 v64.26,29.34
EPD_SO  (via drill 0.3 pad 0.64)
  Top 0.203: v64.52,30.99 64.52,31.37 64.86,31.71 U8.37 67.73,31.71 68.83,30.61 68.83,26.61 v69.34,26.1 | U4.2 17.75,28.48 v17.02,29.21
  Bottom 0.203: v64.52,30.99 64.26,30.99 62.86,29.59 25.91,29.59 24,31.5 21.84,31.5 20.82,30.48 18.28,30.48 v17.02,29.21 | U7.6 69.39,26.05 v69.34,26.1
EPD_STV_IN  (via drill 0.3 pad 0.64)
  Top 0.203: U8.45 65.88,27.69 63.25,27.69 v62.74,28.19 | 24.64,29.46 R15.6 v23.88,29.59
  Bottom 0.203: v23.88,29.59 25.02,28.45 62.48,28.45 v62.74,28.19
EPD_VCL  (via drill 0.3 pad 0.64)
  Top 0.203: v60.83,25.78 60.83,24.77 C23.2
  Bottom 0.203: U7.9 62.07,24.55 v60.83,25.78
EPD_VCOM_PANEL  (via drill 0.3 pad 0.64)
  Top 0.203: R32.1 v60.71,8.76 C21.2 | v69.22,9.14 72.2,12.13 72.2,46.55 69.03,49.72 U8.1 64.7,49.72 v64.13,49.15 64.57,48.72 U8.3
  Top 0.305: C1.1 C2.1 v55.88,48.64 55.88,48.01 R6.2 | R16.3 27.69,40.89 v27.56,41.02
  Bottom 0.203: U7.40 69.31,9.05 v69.22,9.14 | U7.39 69.36,9.55 69.22,9.4 v69.22,9.14 | v69.22,9.14 61.09,9.14 v60.71,8.76
  Bottom 0.305: v64.13,49.15 56.39,49.15 v55.88,48.64 48.26,41.02 v27.56,41.02
EPD_VDH  (via drill 0.3 pad 0.64)
  Top 0.203: v58.55,10.29 57.4,9.14 C19.2 | v68.58,11.3 69.85,11.3 71.06,12.51 71.06,46.16 69.51,47.72 U8.5 63.92,47.72 61.72,49.91 61.72,50.93 60.71,51.94 60.71,52.07 60.58,52.2 C25.1 v60.58,53.47 | v37.59,43.18 Q9.3 41.02,43.18 41.27,42.93
  Top 0.254: 41.27,42.93 41.27,40.9 42.8,39.37 44.16,39.37 47.97,35.56 49.53,35.56 T_VDH.T
  Bottom 0.203: v58.55,10.29 59.31,11.05 60.96,11.05 61.34,11.43 68.45,11.43 v68.58,11.3 68.84,11.05 U7.36 | v60.58,53.47 57.15,50.04 55.24,50.04 47.5,42.29 38.48,42.29 v37.59,43.18
EPD_VDL  (via drill 0.3 pad 0.64)
  Top 0.203: v58.55,6.98 57.4,6.98 C20.2 | v68.07,10.54 69.6,10.54 71.44,12.38 71.44,46.29 69.51,48.22 U8.4 64.05,48.22 62.36,49.91 62.36,52.07 C24.1 v62.61,53.47 | R16.7 v31.37,41.66 Q11.2 | 32.51,40.26 Q11.2 | 32.77,40.26 Q11.2
  Top 0.254: T_VDL.T 48.26,42.04 v48.89,42.67
  Bottom 0.203: U7.37 68.2,10.55 | 68.2,10.55 59.7,10.55 58.55,9.4 v58.55,6.98 | v62.61,53.47 58.8,49.66 55.88,49.66 v48.89,42.67 47.88,41.66 v31.37,41.66 | v68.07,10.54 68.19,10.54 68.2,10.55
EPD_VGH  (via drill 0.3 pad 0.64)
  Top 0.203: v58.17,12.32 57.4,13.08 C17.2 | 65.91,26.23 U8.48 65.97,26.21 65.98,26.23 67.31,26.23 | 60.58,48.01 61.87,46.72 U8.7 69.49,46.72 70.3,45.91 70.3,25.97 69.85,25.53 69.09,25.53 68.39,26.23 67.69,26.23 | C27.1 v61.47,48.26 | v66.04,12.7 66.93,12.7 67.49,13.26 67.49,26.21 67.5,26.23 | 67.31,26.23 67.5,26.23 | 67.69,26.23 67.5,26.23 | 67.31,26.23 67.5,26.04 67.69,26.23 | Q8.3 42.29,41.02 42.99,40.32 v43.94,40.32
  Top 0.254: v43.94,40.32 44.77,40.32 T_VGH.T
  Top 0.305: 60.58,48.01 C27.1
  Bottom 0.203: U7.34 69.49,12.05 68.83,12.7 v66.04,12.7 61.34,12.7 60.71,12.06 58.42,12.06 v58.17,12.32 | v61.47,48.26 56.39,48.26 48.45,40.32 v43.94,40.32
EPD_VGL  (via drill 0.3 pad 0.64)
  Top 0.203: 57.4,11.3 C18.2 57.53,11.3 v58.55,11.3 | 70.67,25.33 70.67,46.04 69.5,47.22 U8.6 63.53,47.22 63.31,47.44 | 70.67,25.33 70.67,25.15 | 70.67,25.15 70.67,24.96 | v68.07,12.06 70.1,12.06 70.67,12.63 70.67,24.9 70.67,24.96 | U8.47 64.56,26.71 v64.52,26.67 | C26.1 60.83,50.04 60.83,49.91 63.31,47.44 | 70.48,25.15 68.58,25.15 v68.07,25.65 | 70.48,25.15 70.67,25.15 | v63.31,47.37 63.31,47.44 | 70.67,25.33 70.48,25.15 | 70.67,24.96 70.48,25.15
  Top 0.254: T_VGL.T v50.8,40.64
  Top 0.305: C16.2 v47.88,14.99
  Top 0.61: C16.2 45.09,14.99 D5.+
  Bottom 0.203: U7.35 69.35,11.55 68.83,12.06 v68.07,12.06 61.34,12.06 60.83,11.56 58.8,11.56 v58.55,11.3 | v63.31,47.37 62.93,46.99 57.15,46.99 v50.8,40.64 | v68.07,25.65 67.44,25.65 66.42,26.67 v64.52,26.67
  Bottom 0.305: v58.55,11.3 51.56,11.3 v47.88,14.99
GND  (via drill 0.3 pad 0.64)
  Top 0.203: U8.8 68.08,46.22 v68.58,45.72 | 37.85,29.59 37.85,28.83 | 37.85,28.83 37.85,28.19 37.59,27.94 37.02,27.94 R21.1 | R21.3 37.85,29.59 | R21.2 37.85,28.83 | U8.40 64.27,30.21 63.88,30.61 63.88,31.83 64.27,32.22 U8.36 67.14,32.22 | 72.39,47.88 72.39,46.99 72.64,46.74 72.64,8.25 | R21.4 37.66,30.42 37.85,30.23 37.85,29.59
  Top 0.305: U3.13 6.32,42.39 v5.97,42.04
  Top 0.406: U4.13 17.75,33.5 C22.1
  Bottom 0.203: U7.33 71.98,12.55 | U7.3 69.52,27.55 v69.44,27.62 | 72.39,47.88 72.39,32.64 72.66,32.37 72.66,24.65
  other vias: 5.21,48.01 8.25,42.42 10.79,44.2 10.79,43.18 19.05,42.93 5.84,39.88 8.64,39.62 50.8,9.52 52.07,51.44 46.99,9.52 50.16,51.44 68.58,43.81 68.58,41.27 68.58,38.73 68.58,35.56 40,34.92 41.27,34.92 34.92,31.37 36.96,31.37 29.21,22.23 46.99,12.7 34.92,20.95 38.1,20.95 40.64,20.95 31.11,37.47 29.21,37.47 26.03,13.72 31.75,13.72 39.88,13.72 23.49,22.23 25.4,22.23 62.86,5.08 65.41,5.08 69.6,31.62 46.99,2.54 64.13,3.81 66.67,3.81 26.67,26.92 27.3,33.02 26.03,33.02 31.18,31.05 30.48,27.3 19.68,23.5 20.95,23.5 20.95,28.19 20.95,29.21 22.35,42.93 23.24,32.38 25.27,26.92 23.88,26.92 69.6,29.84 20.32,42.93 20.32,47.62 19.05,47.62 15.88,47.62 10.79,24.13 35.18,25.4 38.1,25.4 13.34,36.83 17.14,36.83 14.73,40.26 46.99,4.57 48.13,4.57 55.5,4.57 57.15,2.54 20.32,34.29 20.32,35.56 32.38,27.3 5.77,10.79 10.85,10.79 10.78,22.23 5.77,19.05 22.28,2.54 22.28,5.71 50.85,20.95 50.85,18.41 47.68,20.95 50.85,23.5 47.68,23.5 44.5,23.5 3.23,23.5 1.32,23.5 26.72,52.7 14.66,53.34 9.58,53.34 19.74,53.34 36.25,53.34 47.04,53.34 17.83,10.79 17.83,12.06 51.49,35.56 45.77,31.75 45.77,35.56 49.58,38.1 1.32,48.26 1.32,45.72 1.32,43.18 1.32,40.64 1.32,37.47 1.32,34.29 3.86,2.54 3.86,5.71 34.04,13.72 37.21,13.72 43.18,15.88 34.92,1.91 38.1,34.92 15.86,18.41
  pour Bottom (isolate 0.254): 0,0 73.03,0 73.03,54.61 0,54.61
  pour Top (isolate 0.254): 0,0 73.03,0 73.03,54.61 0,54.61
M_/EPD_CS  (via drill 0.3 pad 0.64)
  Top 0.203: J4.3 v33.91,49.78
  Top 0.406: U4.12 18.4,33.01 v18.54,33.15
  Bottom 0.203: v18.54,33.15 18.67,33.02 22.61,33.02 23.75,34.16 23.75,47.85 25.68,49.78 v33.91,49.78
M_/SD_CS  (via drill 0.3 pad 0.64)
  Top 0.203: U3.12 6.97,42.08 7.58,41.47 10.35,41.47 12.06,43.18 v17.14,43.18 | v19.68,31.24 19.68,32.12 U4.10 | R20.6 15.18,26.92 v15.75,27.5
  Top 0.305: J3.5 v17.14,50.8
  Bottom 0.203: v17.14,50.8 v17.14,43.18 17.14,40.26 15.75,38.86 15.75,31.24 | v15.75,27.5 15.75,31.24 | v19.68,31.24 15.75,31.24
M_/WORD_STOCK_CS  (via drill 0.3 pad 0.64)
  Top 0.203: v19.05,28.07 U4.4 19.05,25.4 18.8,25.15 16.79,25.15 16.51,25.43 16.51,27.56 16,28.07 14.73,28.07 14.35,27.69 R20.7 | 22.48,37.34 22.35,37.47 | D4.- 21.59,37.08 21.59,35.56 22.48,34.67 22.48,27.18 v22.73,26.92 | v29.97,49.15 31.37,49.15 J4.2
  Top 0.305: v25.4,37.47 22.35,37.47 D4.-
  Bottom 0.203: v29.97,49.15 26.03,49.15 25.4,48.51 v25.4,37.47 | v22.73,26.92 21.08,26.92 19.94,28.07 v19.05,28.07
M_CKV  (via drill 0.3 pad 0.64)
  Top 0.203: R21.7 34.16,28.83 33.66,28.32 33.66,25.81 32.99,25.15 v31.37,25.15 31.11,25.4 31.11,26.27 U6.5
  Top 0.305: 14.6,2.29 14.73,2.16 14.48,1.91 J5.3 14.99,2.29 14.6,2.67 14.6,6.86 13.84,7.62 13.84,23.24 13.34,23.75 v13.34,24.77
  Bottom 0.203: v31.37,25.15 31.11,25.4 16.26,25.4 15.62,24.77 v13.34,24.77
M_EPD_/RESET  (via drill 0.3 pad 0.64)
  Top 0.203: U3.9 8.92,44.42 8.51,44.83 R4.1 9.27,46.36 10.67,46.36 13.08,43.94 v22.22,43.94
  Top 0.305: J3.7 v22.22,50.8
  Bottom 0.203: v22.22,43.94 v22.22,50.8
M_EPD_BORDER
  Top 0.203: R36.1 15.75,46.23 14.6,47.37 J3.4
M_EPD_BUSY  (via drill 0.3 pad 0.64)
  Top 0.305: J3.8 v24.76,47.88
  Bottom 0.203: U7.2 71.61,28.05 71.75,28.19 71.75,32 71.37,32.38 65.02,32.38 62.61,29.97 26.07,29.97 24.13,31.91 24.13,47.24 v24.76,47.88
M_EPD_DISCHARGE
  Top 0.305: R42.2 35.56,46.36 34.29,47.62 29.84,47.62 28.83,48.64 J4.1
M_EPD_PANEL_ON  (via drill 0.3 pad 0.64)
  Top 0.203: J3.3 11.94,52.58 11.94,47.37 13.84,45.47 v22.86,45.47
  Top 0.305: R27.1 v29.21,36.07 | v25.4,36.07 v23.11,36.07
  Bottom 0.203: v23.11,36.07 23.37,36.32 23.37,44.96 v22.86,45.47
  Bottom 0.305: v29.21,36.07 v25.4,36.07
M_EPD_PWM  (via drill 0.3 pad 0.64)
  Top 0.203: v21.59,34.29 22.1,33.78 22.1,21.08 v22.22,20.95
  Top 0.305: J3.6 v21.59,50.16 | v32.77,20.95 32.77,16.76 R29.2
  Top 0.406: Q7.1 34.42,17.02 37.72,17.02 R26.2 | 34.42,16.64 32.89,16.64 32.77,16.76
  Top 0.61: 34.42,16.64 Q7.1
  Bottom 0.203: v21.59,50.16 v21.59,34.29
  Bottom 0.305: v22.22,20.95 v32.77,20.95
M_MISO
  Top 0.305: R12.6 11.68,31.5 | 11.68,31.5 11.43,31.5 | 11.43,31.5 11.18,31.5 | 11.18,31.5 8.64,31.5 | R12.8 11.62,29.91 11.43,30.1 11.43,30.48 | 11.43,30.48 11.43,30.73 | 11.43,30.73 11.43,30.99 | 11.43,30.99 11.43,31.24 | 11.43,31.24 11.43,31.5 | R12.7 11.68,30.73 | 11.68,30.73 11.43,30.73 | 11.68,31.5 11.43,31.24 | 11.43,31.24 11.18,31.5 | 11.43,30.99 11.68,30.73 | 11.68,30.73 11.43,30.48
  Top 0.61: 8.64,31.5 J7.6
M_MOSI
  Top 0.305: U3.2 6.32,35.78 R3.1 | R3.1 6.1,35.43 | J7.2 5.08,28.57 5.4,28.89 5.4,32.45 6.97,34.02 6.97,34.69 R3.1
M_OE123  (via drill 0.3 pad 0.64)
  Top 0.203: J5.2 17.14,5.33 16.76,5.71 16.64,5.71 | U6.2 29.18,25.18 29.84,24.51 v30.48,24.51 32.93,24.51 34.04,25.62 34.04,27.69 34.35,28 R21.8
  Top 0.305: 17.14,4.83 J5.2 | v13.97,24.13 14.35,23.75 14.35,8 16.64,5.71
  Bottom 0.203: v30.48,24.51 29.97,25.02 16.76,25.02 15.88,24.13 v13.97,24.13
M_RESET  (via drill 0.3 pad 0.64)
  Top 0.305: J6.6 v38.73,1.91 | v53.21,3.81 54.1,3.81 SW1.2 | v59.31,3.81 60.2,2.92 60.26,2.92 RST.2
  Bottom 0.305: v38.73,1.91 40.64,3.81 v53.21,3.81 v59.31,3.81
M_SCK
  Top 0.305: U3.5 8.27,35.8 R37.1 7.62,34.67 7.62,33.78 6.04,32.2 6.04,28.88 6.35,28.57 J7.5
M_STV_IN  (via drill 0.3 pad 0.64)
  Top 0.203: U6.9 31.78,33.05 32,33.27 33.4,33.27 33.66,33.02 33.66,30.1 34.16,29.59 R21.6 36.07,29.59 36.2,29.46 36.2,27.56 35.94,27.3 34.67,27.3 34.42,27.05 34.42,25.44 32.85,23.88 29.59,23.88 v29.34,24.13 | J5.4 12.06,5.08
  Top 0.305: 12.06,5.33 12.06,5.08 11.94,5.08 | J5.4 12.06,6.35 13.34,7.62 13.34,22.86 v12.7,23.5
  Bottom 0.203: v29.34,24.13 28.83,24.64 17.27,24.64 16.13,23.5 v12.7,23.5
M_TEMP_SEN  (via drill 0.3 pad 0.64)
  Top 0.203: v52.7,26.67 52.7,28.19 C56.2
  Top 0.254: U9.4 49.93,29.23 R23.2 C56.2
  Top 0.305: J5.1 v19.68,3.81
  Bottom 0.203: v19.68,3.81 19.68,20.83 22.35,23.5 30.61,23.5 34.04,26.92 52.45,26.92 v52.7,26.67
M_VCC_3V3
  Top 0.61: Q5.3 44.45,9.14 43.18,7.87 37.46,7.87 34.92,5.33 J6.5
M_VCC_5V
  Top 0.61: J6.4 32.38,5.71 36.83,10.16 D3.+
  Top 0.813: R19.1 R14.2 D3.+
N$1
  Top 0.305: R2.1 44,1.14 PWR.2
N$2
  Top 0.61: Q5.1 40.89,11.94 R19.2
N$3
  Top 0.61: D5.- D6.+ 40.77,17.53 C15.2
N$4
  Top 0.61: Q7.2 34.42,15.11 R29.1 R30.1 29.97,15.11 D7.- 28.96,14.1
N$6
  Top 0.203: R27.2 R28.2 42.04,37.59 Q2.1
N$7
  Top 0.305: U3.11 7.62,44.83 R11.1
N$8
  Top 0.406: U2.3 32.64,11.43 D3.- 34.8,11.05 C30.2
N$9
  Top 0.406: R26.1 37.21,15.11 Q7.3
  Top 0.61: C15.1 38.23,14.99 R26.1
N$10
  Top 0.203: R42.1 R39.2 39.88,44.2 40,44.07 40.13,44.07 | 40.13,44.07 Q8.1 | Q9.1 36.45,44.45 40,44.45 40.13,44.32 40.13,44.07
N$11
  Top 0.203: R25.2 40.13,33.91 Q3.1 42.42,33.91 44.2,35.69 Q2.3
N$12
  Top 0.203: R32.2 R31.1
N$13
  Top 0.203: 28.51,42.48 R16.1 29.15,43.18 34.04,43.18 34.67,43.81 Q10.3
N$14
  Top 0.305: R36.2 32.38,46.23 arc-90 Q10.1
N$15
  Top 0.203: U8.14 64.42,43.22 64.26,43.05 54.86,43.05 54.1,42.29 C4.1
N$16
  Top 0.203: R18.2 36.7,42.04 | 36.7,42.04 36.7,42.29 Q9.2 | Q8.2 40.26,41.91 39.75,41.91 39.62,41.78 36.83,41.78 36.83,41.91 36.7,42.04
N$19
  Top 0.203: U6.12 29.83,33.26 30.23,33.66 33.53,33.66 34.04,33.15 34.04,30.86 34.48,30.42 R21.5
N$20
  Top 0.203: U4.3 18.4,28.97 17.53,29.84 14.16,29.84 R12.1
N$21
  Top 0.203: 14.22,30.61 R12.2 14.86,30.73 15.37,30.23 17.8,30.23 20.35,27.68 U4.6 20.32,26.32
N$22
  Top 0.203: U4.8 21.05,31.08 20.57,30.61 15.62,30.61 14.73,31.5 R12.3
N$23
  Top 0.203: R15.1 29.27,28 29.83,27.45 U6.3
N$24
  Top 0.203: R15.3 30.99,29.59 32.48,31.08 U6.8
N$25
  Top 0.203: R15.4 29.91,30.42 30.48,30.99 U6.11
N$26
  Top 0.203: R15.2 30.48,28.83 31.78,27.53 U6.6
N$27
  Top 0.203: U4.11 19.05,31.24 18.92,31.11 15.88,31.11 14.67,32.32 R12.4
N$28
  Top 0.203: Q11.1 32.32,42.48 R16.8 29.53,42.48 28.7,41.66 R16.2
N$30
  Top 0.203: R1.2 R6.1
N$34  (via drill 0.3 pad 0.64)
  Top 0.203: C34.1 55.63,25.02 56.52,25.91 v59.05,25.91
  Bottom 0.203: U7.10 61.55,24.05 59.69,25.91 v59.05,25.91
N$35  (via drill 0.3 pad 0.64)
  Top 0.203: v58.42,25.27 57.53,25.27 57.4,25.15 C34.2
  Bottom 0.203: U7.11 61.42,23.55 59.69,25.27 v58.42,25.27
N$36  (via drill 0.3 pad 0.64)
  Top 0.203: C39.1 62.48,22.73 61.59,23.62 60.2,23.62 v59.56,24.26
  Bottom 0.203: U7.12 60.77,23.05 v59.56,24.26
N$37  (via drill 0.3 pad 0.64)
  Top 0.203: C39.2 60.71,22.73 60.2,23.24 v59.69,23.24
  Bottom 0.203: U7.13 60.38,22.55 v59.69,23.24
N$39
  Top 0.203: U8.15 65.91,42.67 56.26,42.67 55.88,42.29 C4.2
N$40
  Top 0.203: U8.12 64.41,44.22 64.01,43.81 56.52,43.81 56.13,44.2 56.13,44.32 C3.1
N$41
  Top 0.203: U8.17 60.64,41.72 60.58,41.66 C31.2
N$42
  Top 0.203: U8.16 59.61,42.22 58.8,41.4 C31.1
N$43
  Top 0.203: U8.18 62.3,41.22 61.28,40.2 57.47,40.2 56.64,41.02 54.86,41.02 54.23,40.39 54.23,40.13 C8.1
N$44
  Top 0.203: U8.19 62.3,40.72 61.41,39.81 56.07,39.81 C8.2
N$45
  Top 0.203: U8.21 62.32,39.72 61.59,38.99 60.58,38.99 C33.2
N$46
  Top 0.203: U8.20 62.31,40.22 61.53,39.43 59.5,39.43 58.93,38.86 58.93,38.61 C33.1
N$47
  Top 0.203: U8.22 63.09,39.22 61.34,37.47 56.01,37.47 55.88,37.59 C5.1
N$48
  Top 0.203: U8.23 63.23,38.72 61.47,36.96 54.86,36.96 54.1,37.72 C5.2
N$49
  Top 0.203: U8.24 63.36,38.22 61.72,36.58 54.99,36.58 54.1,35.69 C7.1
N$50
  Top 0.203: U8.25 63.5,37.72 61.98,36.2 56.39,36.2 55.88,35.69 C7.2
N$51
  Top 0.203: U8.26 63.63,37.22 62.23,35.81 59.56,35.81 58.8,35.05 C36.1
N$52
  Top 0.203: U8.27 63.77,36.72 62.36,35.31 60.58,35.31 C36.2
N$53
  Top 0.203: U8.28 63.9,36.22 61.47,33.78 57.28,33.78 56.64,34.42 54.86,34.42 54.1,33.66 C9.1
N$54
  Top 0.203: U8.29 64.04,35.72 61.72,33.4 C9.2
N$55
  Top 0.203: U8.30 64.17,35.22 61.98,33.02 59.56,33.02 58.8,32.26 C38.1
N$56
  Top 0.203: U8.31 64.31,34.72 62.1,32.51 60.58,32.51 C38.2
N$57
  Top 0.203: U8.32 64.44,34.22 61.21,30.99 56.26,30.99 C6.1
N$58
  Top 0.203: U8.11 64.4,44.72 63.88,44.2 57.91,44.2 R1.1
N$67
  Top 0.203: U8.43 63.36,28.71 62.48,29.59 60.58,29.59 R17.1
N$74
  Top 0.305: U3.3 6.97,39 8.99,41.02 11.43,41.02 arc90 R8.1
N$76
  Top 0.305: R10.1 9.52,39.37 8.92,38.77 U3.6
N$80
  Top 0.305: U3.8 9.62,45.05 R9.1
N$81  (via drill 0.3 pad 0.64)
  Top 0.203: C35.1 55.63,22.73 56.52,23.62 v58.93,23.62
  Bottom 0.203: U7.14 59.87,22.05 59.05,22.86 59.05,23.5 v58.93,23.62
N$82
  Top 0.203: U8.13 64.42,43.72 64.13,43.43 54.99,43.43 54.1,44.32 C3.2
N$85  (via drill 0.3 pad 0.64)
  Top 0.203: 57.4,22.35 C35.2 57.4,22.73 57.53,22.86 v58.42,22.86
  Bottom 0.203: U7.15 59.73,21.55 v58.42,22.86
N$87
  Top 0.305: R5.2 60.14,1.14 RST.1
N$88  (via drill 0.3 pad 0.64)
  Top 0.203: v59.05,21.34 61.59,21.34 62.36,20.57 62.36,20.32 C32.1
  Bottom 0.203: U7.16 59.34,21.05 v59.05,21.34
N$89  (via drill 0.3 pad 0.64)
  Top 0.203: v58.55,20.57 60.71,20.57 C32.2
  Bottom 0.203: U7.17 58.57,20.55 v58.55,20.57
N$90  (via drill 0.3 pad 0.64)
  Top 0.203: 57.53,19.68 57.4,19.81 57.4,19.94 | 57.4,19.94 C37.1 | v59.18,19.94 57.4,19.94
  Bottom 0.203: U7.18 59.29,20.05 v59.18,19.94
N$91  (via drill 0.3 pad 0.64)
  Top 0.203: v59.31,19.05 56.52,19.05 55.63,19.94 C37.2
  Bottom 0.203: U7.19 59.8,19.55 v59.31,19.05
N$92  (via drill 0.3 pad 0.64)
  Top 0.203: v59.69,18.29 60.58,18.29 60.71,18.16 C10.1
  Bottom 0.203: U7.20 60.45,19.05 v59.69,18.29
N$93  (via drill 0.3 pad 0.64)
  Top 0.203: C10.2 62.48,17.65 61.59,16.76 60.2,16.76 v58.55,18.41
  Bottom 0.203: U7.21 60.84,18.55 59.94,17.65 59.31,17.65 v58.55,18.41
N$94  (via drill 0.3 pad 0.64)
  Top 0.203: v58.55,17.53 57.78,17.53 | 57.78,17.53 57.66,17.53 | C11.1 57.78,17.53
  Bottom 0.203: U7.22 60.84,18.05 60.07,17.27 58.8,17.27 v58.55,17.53
N$95  (via drill 0.3 pad 0.64)
  Top 0.203: 55.75,17.65 55.75,17.4 55.88,17.4 | 55.88,17.4 56.52,16.76 59.05,16.76 v59.18,16.64 | C11.2 55.63,17.65 55.88,17.4
  Bottom 0.203: U7.23 61.11,17.55 60.2,16.64 v59.18,16.64
N$96  (via drill 0.3 pad 0.64)
  Top 0.203: v59.69,16 60.58,16 60.71,15.88 C12.1
  Bottom 0.203: U7.24 61.24,17.05 60.2,16 v59.69,16
N$97  (via drill 0.3 pad 0.64)
  Top 0.203: C12.2 62.36,15.49 62.36,15.24 61.59,14.48 60.07,14.48 v58.55,16
  Bottom 0.203: U7.25 61.38,16.55 60.2,15.37 59.18,15.37 v58.55,16
N$98  (via drill 0.3 pad 0.64)
  Top 0.203: C13.1 57.4,15.11 v58.55,15.11
  Bottom 0.203: U7.26 61.51,16.05 60.32,14.86 58.8,14.86 v58.55,15.11
N$99  (via drill 0.3 pad 0.64)
  Top 0.203: C13.2 55.63,15.37 56.52,14.48 58.29,14.48 v58.55,14.22
  Bottom 0.203: U7.27 61.65,15.55 60.45,14.35 58.67,14.35 v58.55,14.22
N$100  (via drill 0.3 pad 0.64)
  Top 0.203: v59.82,13.72 60.45,13.72 60.71,13.46 C14.1
  Bottom 0.203: U7.28 61.78,15.05 60.45,13.72 v59.82,13.72
N$101  (via drill 0.3 pad 0.64)
  Top 0.203: C14.2 62.23,13.08 62.23,12.83 61.59,12.19 60.32,12.19 v58.99,13.53
  Bottom 0.203: U7.29 61.92,14.55 60.45,13.08 59.44,13.08 v58.99,13.53
S_MOSI  (via drill 0.3 pad 0.64)
  Top 0.203: U8.38 67.72,31.21 68.45,30.48 68.45,27.3 67.94,26.8 v67.31,26.8 | J2.3 15.29,15.19 14.86,15.62 14.86,25.15 v15.24,25.53
  Top 0.305: R8.2 v14.22,41.27 15.43,41.27 U5.6
  Bottom 0.203: 15.24,25.78 32.38,25.78 33.91,27.3 61.21,27.3 61.8,26.72 63.55,26.72 64.26,27.43 66.42,27.43 67.06,26.8 v67.31,26.8 67.69,26.8 67.82,26.67 69.6,26.67 69.72,26.54 U7.5 | 15.24,25.78 11.68,25.78 10.41,27.05 10.41,40.2 10.73,40.51 13.46,40.51 v14.22,41.27 | v15.24,25.53 15.24,25.78
S_SCK  (via drill 0.3 pad 0.64)
  Top 0.203: U5.1 15.56,39.31 15.62,39.37 | U8.39 67.71,30.71 68.07,30.35 68.07,27.81 v67.82,27.56 | v15.88,26.35 15.88,25.27 15.24,24.64 15.24,18.16 16.01,17.39 J2.5
  Top 0.305: R10.2 v14.22,39.37 15.62,39.37 15.62,39.18 U5.1
  Bottom 0.203: 15.88,26.16 32.26,26.16 33.78,27.69 61.47,27.69 62.01,27.14 63.33,27.14 64.01,27.81 66.55,27.81 66.93,27.43 67.82,27.43 | 15.88,26.16 11.89,26.16 10.79,27.25 10.79,40 10.92,40.13 11.18,40.13 11.3,40 11.3,38.73 11.43,38.61 11.68,38.61 11.81,38.73 11.81,40 11.94,40.13 12.19,40.13 12.32,40 12.32,38.73 12.45,38.61 12.7,38.61 12.83,38.73 12.83,40 12.95,40.13 13.21,40.13 13.34,40 13.34,38.73 13.46,38.61 14.1,38.61 14.22,38.73 v14.22,39.37 | 15.88,26.16 v15.88,26.35 | 67.82,27.43 67.94,27.43 68.33,27.05 U7.4 | v67.82,27.56 67.82,27.43
SD_DO
  Top 0.203: U4.9 20.35,32.92 20.7,33.27 21.44,33.27 21.72,33 21.72,21.43 19.87,19.59 J2.7
VCC_3V3  (via drill 0.3 pad 0.64)
  Top 0.203: 17.46,41.81 U5.4 17.4,41.46 | 19.56,41.15 C42.2 | Q3.2 42.29,32.13 43.18,33.02 43.18,33.78 43.69,34.29
  Top 0.254: 43.69,34.29 T_3V3.T
  Top 0.305: U6.14 28.48,34.29 C47.2 | C43.2 30.23,44.45 32.26,44.45 32.51,44.2 Q10.2 | R13.2 21.21,39.75 26.42,39.75 | 26.42,39.75 26.67,39.75 | 26.42,39.75 26.67,40 | 26.42,39.75 26.67,39.5 | R13.2 21.08,39.5 19.81,38.23 19.81,36.2 19.18,35.56 18.16,35.56 16.89,34.29 | R13.2 21.08,39.75 C42.2 | 17.4,41.46 17.4,42.29 17.14,42.55 14.6,42.55 v14.22,42.16 | 29.21,16.64 29.21,17.4 D7.+ | 48.89,5.97 48.89,5.71
  Top 0.406: U4.14 17.05,34.26 C22.2 16.89,34.29 R24.1 | U3.14 5.62,45.18 C40.2 4.32,45.59 3.81,46.1 3.81,48.13 4.57,48.89 7.62,48.89 v8.51,48.01 R4.2 | U5.4 19.43,41.4 C42.2 | C41.2 R25.1 42.04,32.26 Q3.2 | C45.2 25.4,20.12 28.65,23.37 42.8,23.37 | C29.+ 23.37,12.89 | 23.37,12.89 24.7,12.89 R40.1 | C28.2 23.49,13.02 23.37,12.89 | C28.2 23.3,15.11 21.78,16.64 C44.2 21.24,16.29 J2.4 | C28.2 23.75,15.11 25.27,16.64 C45.2 | C45.2 C49.2 29.21,16.64 R30.2 | C43.2 28.83,43.56 27.43,43.56 26.67,42.8 26.67,40 26.67,39.75 26.67,39.5 26.67,36.45 28.7,34.42 C47.2 33.66,34.29 35.69,32.26 C41.2 | 42.8,23.37 43.05,23.37 | 43.05,23.37 43.18,23.37 | 43.05,23.62 R22.1 C48.2 40.96,27.81 39.43,29.34 C46.2 39.12,29.46 39.12,29.65 38.1,30.67 C41.2 | 43.05,23.5 43.05,23.37 | 43.05,23.62 42.8,23.37 | 43.18,23.37 48.89,17.65 48.89,5.97 | 48.64,5.71 48.89,5.71 49.15,5.71 | 48.64,5.71 46.67,5.71 46.29,5.33 PWR.1 | 49.15,5.71 55.37,5.71 55.75,5.33 R5.1 | 48.89,5.97 48.64,5.71 | 48.89,5.97 49.15,5.71 | 43.05,23.62 43.05,23.5 | 43.05,23.5 43.18,23.37
  Bottom 0.305: v14.22,42.16 10.41,42.16 8.51,44.07 v8.51,48.01
VCC_3V3_EPD  (via drill 0.3 pad 0.64)
  Top 0.203: U8.10 64.77,45.22 v64.52,45.47 64.77,45.72 U8.9 | U8.49 64.58,25.71 62.74,27.56 61.09,27.56 R17.2
  Top 0.254: Q3.3 46.99,33.02 T_E3V3.T
  Top 0.305: R17.2 58.93,29.84 59.56,30.48 61.59,30.48 v64.13,33.02 | v44.2,31.88 Q3.3 | U8.49 66.87,25.71 67.06,25.53 67.06,18.29 C50.2 C51.2 v66.67,13.33 | v64.52,45.47 64.01,44.96 C53.2 C52.2
  Bottom 0.203: U7.32 69.5,13.05 69.22,13.33 69.43,13.55 U7.31
  Bottom 0.305: 69.22,13.33 v66.67,13.33 | v64.52,45.47 64.52,33.4 v64.13,33.02 61.98,30.86 45.21,30.86 v44.2,31.88
VCC_OUT  (via drill 0.38 pad 0.81)
  Top 0.61: R40.2 25.53,10.54 C54.1 | Q5.2 v42.42,8.89 | C54.1 U2.2 | C54.1 27.94,9.52 v28.57,8.89
  Bottom 0.61: v42.42,8.89 v28.57,8.89
VCOM_DRIVER  (via drill 0.3 pad 0.64)
  Top 0.203: R31.2 60.71,11.56 60.07,11.56 v58.93,12.7
  Bottom 0.203: U7.30 62.05,14.05 60.71,12.7 v58.93,12.7
VDD
  Top 0.305: R22.2 43.18,29.46 C55.1 45.2,29.23 U9.1
WS_DO  (via drill 0.3 pad 0.64)
  Top 0.203: U5.5 v16.51,40.51 | U4.5 v19.7,27.18 v19.68,27.18
  Bottom 0.203: v19.68,27.18 19.43,26.92 15.4,26.92 15.04,27.28 15.04,39.04 v16.51,40.51

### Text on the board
tPlace: D7 | D13 | D0 | D8 | GND | NC | MISO | MOSI | SCK | NC | GND | A0 | GND | 5V | RESET | A5 | VIN | GND | 3V3
bPlace: Small e-Paper Shield | v2.2 04/30/2014 | by Seeed Studio | www.seeedstudio.com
